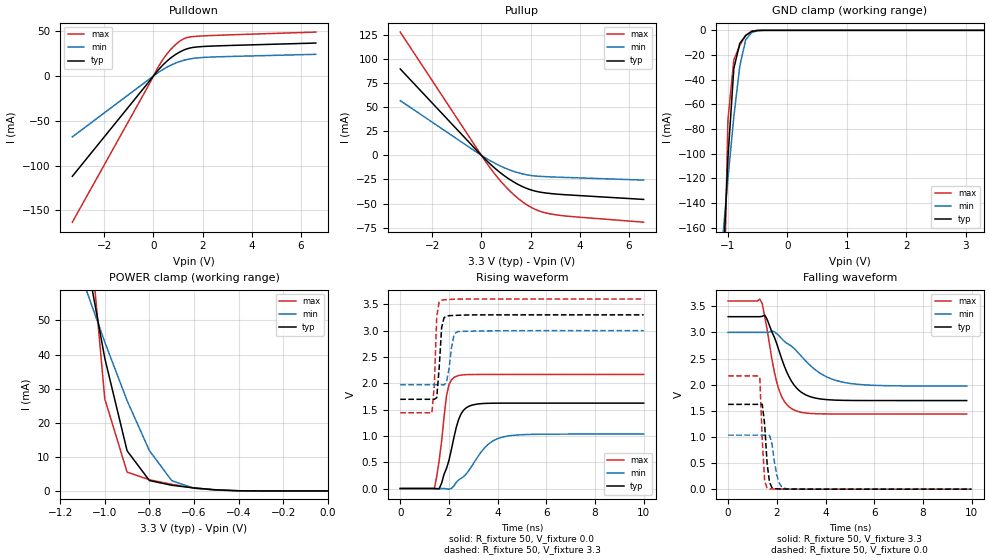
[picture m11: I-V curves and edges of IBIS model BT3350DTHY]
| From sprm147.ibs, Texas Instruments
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[Model]   BT3350DTHY
Model_type   I/O
Vinh = 2.00
Vinl = 0.80
Enable   Active-Low
Polarity   Non-Inverting
| signals   A, GZ, Y
Vmeas = 1.5
|   typ   min   max
C_comp   1.2534194p   1.2234995p   1.2884204p
|   typ   min   max
[Temperature Range]   25   -40   125
|   typ   min   max
[Voltage Range]   3.30V   3.00V   3.60V
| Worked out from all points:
|   slope of the pulldown table from 0 to 0.495 V, typ, clamps not added: 32.6 ohm
|   slope of the pullup table from 0 to 0.495 V, typ, clamps not added: 40.8 ohm
|   GND clamp passes 1 mA (typ) near -0.60 V on its own axis
|   POWER clamp passes 1 mA (typ) near -0.62 V on its own axis
|   rising waveform, R_fixture 50, V_fixture 0.0: 20-80 % time 542ps typ, 1.04ns min, 327ps max; typ from 0 V to 1.62 V
|   falling waveform, R_fixture 50, V_fixture 3.3: 20-80 % time 847ps typ, 1.53ns min, 555ps max; typ from 3.3 V to 1.7 V
|   rising waveform, R_fixture 50, V_fixture 3.3: 20-80 % time 139ps typ, 191ps min, 109ps max; typ from 1.7 V to 3.3 V
|   falling waveform, R_fixture 50, V_fixture 0.0: 20-80 % time 161ps typ, 227ps min, 131ps max; typ from 1.62 V to 0 V
[Pulldown]
|   Voltage   I(typ)   I(min)   I(max)
-3.3V     -111.9mA   -67.94mA   -163.1mA
-200mV    -7.006mA   -4.134mA   -10.54mA
200mV     6.741mA    3.927mA    10.24mA
400mV     12.65mA    7.43mA     18.97mA
600mV     17.74mA    10.51mA    26.32mA
1V        25.63mA    15.38mA    37.32mA
1.3V      29.62mA    17.92mA    42.23mA
1.7V      32.11mA    19.89mA    44.11mA
2.7V      33.64mA    21.42mA    45.44mA
6.6V      36.69mA    24.11mA    48.91mA
[GND_clamp]
|   Voltage   I(typ)   I(min)   I(max)
-3.3V     -3.12A     -1.528A    -8.251A
-1.1V     -211.9mA   -175.7mA   -299.9mA
-1V       -104.1mA   -120.7mA   -73.01mA
-900mV    -30.88mA   -70.06mA   -23.93mA
-800mV    -10.59mA   -29mA      -12.16mA
-700mV    -4.13mA    -7.527mA   -4.074mA
-600mV    -906uA     -1.794mA   -579.2uA
-500mV    -93.04uA   -329.8uA   -34.38uA
-400mV    -5.843uA   -41.9uA    -1.039uA
3.3V      222pA      7.352uA    0A
[Pullup]
|   Voltage   I(typ)   I(min)   I(max)
-3.3V     89.4mA     56.63mA    127.6mA
300mV     -7.585mA   -4.679mA   -11.03mA
700mV     -16.55mA   -10.12mA   -24.18mA
1V        -22.37mA   -13.58mA   -32.81mA
1.6V      -31.52mA   -18.75mA   -46.77mA
1.9V      -34.77mA   -20.4mA    -52.01mA
2.2V      -37.1mA    -21.41mA   -56.04mA
2.5V      -38.56mA   -21.93mA   -58.84mA
2.9V      -39.76mA   -22.41mA   -61.06mA
3.7V      -41.23mA   -23.12mA   -63.43mA
6.6V      -45.64mA   -25.63mA   -69.21mA
[POWER_clamp]
|   Voltage   I(typ)   I(min)   I(max)
-3.3V     1.007A     508.7mA    2.351A
-1.1V     74.68mA    62.06mA    99.72mA
-1V       38.92mA    43.68mA    27.01mA
-900mV    11.77mA    26.47mA    5.519mA
-800mV    3.047mA    11.81mA    3.279mA
-700mV    1.667mA    3.018mA    1.923mA
-600mV    872uA      765.6uA    893.9uA
-500mV    320uA      255.2uA    245.8uA
-400mV    56uA       56.73uA    23.4uA
0V        1pA        1pA        1pA
[Ramp]
|   I(typ)   I(min)   I(max)
dV/dt_r   0.973/0.538n   0.620/1.033n   1.300/0.327n
dV/dt_f   0.963/0.842n   0.616/1.520n   1.297/0.552n
[Rising Waveform]
R_fixture = 50
V_fixture = 0.0
|  pu_on
|  TIME   V(typ)   V(min)   V(max)
0s        18nV       188nV      1nV
1.4ns     396.3uV    -2.314uV   -4.88mV
1.6ns     -5.745mV   -23.07uV   535.5mV
1.9ns     381.5mV    -5.999mV   1.759V
2ns       533.2mV    -12.51mV   1.973V
2.3ns     1.159V     116.3mV    2.133V
2.8ns     1.558V     329.4mV    2.165V
3.5ns     1.617V     789mV      2.167V
4.2ns     1.622V     977mV      2.167V
10ns      1.622V     1.034V     2.167V
[Falling Waveform]
R_fixture = 50
V_fixture = 3.3
V_fixture_min = 3.0
V_fixture_max = 3.6
|  pd_on
|  TIME   V(typ)   V(min)   V(max)
0s        3.3V       3V         3.6V
1.3ns     3.3V       3V         3.637V
1.4ns     3.307V     3V         3.55V
1.6ns     3.249V     2.999V     3.059V
1.9ns     2.906V     3.009V     2.237V
2.1ns     2.634V     2.928V     1.884V
2.7ns     1.997V     2.696V     1.516V
3.4ns     1.765V     2.356V     1.448V
4.6ns     1.701V     2.059V     1.439V
9.8ns     1.695V     1.973V     1.438V
[Rising Waveform]
R_fixture = 50
V_fixture = 3.3
V_fixture_min = 3.0
V_fixture_max = 3.6
|  pd_off
|  TIME   V(typ)   V(min)   V(max)
0s        1.695V     1.973V     1.438V
1.3ns     1.695V     1.973V     1.435V
1.4ns     1.695V     1.973V     1.961V
1.5ns     1.725V     1.973V     3.276V
1.6ns     2.299V     1.973V     3.548V
1.7ns     3.055V     1.973V     3.579V
1.9ns     3.276V     2.02V      3.589V
2.2ns     3.289V     2.902V     3.597V
2.4ns     3.292V     2.984V     3.599V
10ns      3.3V       3V         3.6V
[Falling Waveform]
R_fixture = 50
V_fixture = 0.0
|  pu_off
|  TIME   V(typ)   V(min)   V(max)
0s        1.622V     1.034V     2.167V
1.3ns     1.622V     1.034V     2.139V
1.4ns     1.623V     1.034V     954mV
1.5ns     1.239V     1.033V     154.7mV
1.6ns     489.9mV    1.035V     22.91mV
1.7ns     130mV      1.029V     6.361mV
1.8ns     30.24mV    868.6mV    3.891mV
2ns       6.048mV    263.3mV    2.214mV
2.3ns     2.752mV    16.58mV    939.8uV
10ns      972nV      2.658uV    231nV
